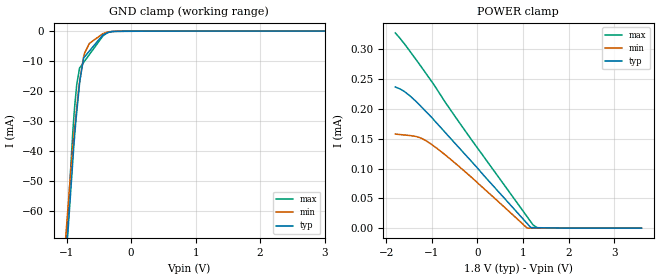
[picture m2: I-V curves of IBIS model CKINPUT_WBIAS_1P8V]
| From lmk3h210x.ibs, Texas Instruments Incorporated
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[Model]   CKINPUT_WBIAS_1P8V
Model_type   Input
Vinl = 0.2
Vinh = 0.4
|   typ   min   max
C_comp   1.5pF   1.4pF   1.6pF
[Voltage Range]   1.8   1.71   1.89
[Temperature Range]   50   125   -40
[Power Clamp Reference]   1.8   1.71   1.89
[GND Clamp Reference]   0   0   0
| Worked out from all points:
|   GND clamp passes 1 mA (typ) near -0.41 V on its own axis
[GND Clamp]
|   Voltage   I(typ)   I(min)   I(max)
-1.8V     -388.2mA   -347.5mA   -421.6mA
-1.003V   -74.18mA   -65.35mA   -69.68mA
-930mV    -51.09mA   -44.88mA   -42.65mA
-877.4mV  -35.11mA   -32.43mA   -25.38mA
-844.7mV  -27.11mA   -25.63mA   -17.87mA
-800.4mV  -17.48mA   -16.99mA   -12.34mA
-737.3mV  -8.951mA   -8.558mA   -10.47mA
-723.4mV  -8.592mA   -7.384mA   -10.05mA
-648.8mV  -6.671mA   -4.121mA   -7.843mA
-440.4mV  -1.313mA   -871.8uA   -1.664mA
-240.3mV  -93.53uA   -80.96uA   -100.1uA
3.6V      0A         0A         0A
[POWER Clamp]
|   Voltage   I(typ)   I(min)   I(max)
-1.8V     237uA      157.9uA    327.8uA
-1.599V   229.3uA    156.4uA    309.3uA
-1.303V   209.5uA    153uA      278.6uA
-1.191V   200.8uA    149.5uA    266.6uA
-1.025V   187.8uA    141.7uA    248.7uA
-702.6mV  160.4uA    122.9uA    211.2uA
-260mV    123uA      94.2uA     162.6uA
1.094V    7.643uA    23.7nA     18.96uA
1.172V    987.3nA    15.94nA    10.68uA
1.219V    925.1nA    11.24nA    5.671uA
1.327V    782.3nA    477.3pA    0A
3.6V      0A         0A         0A
